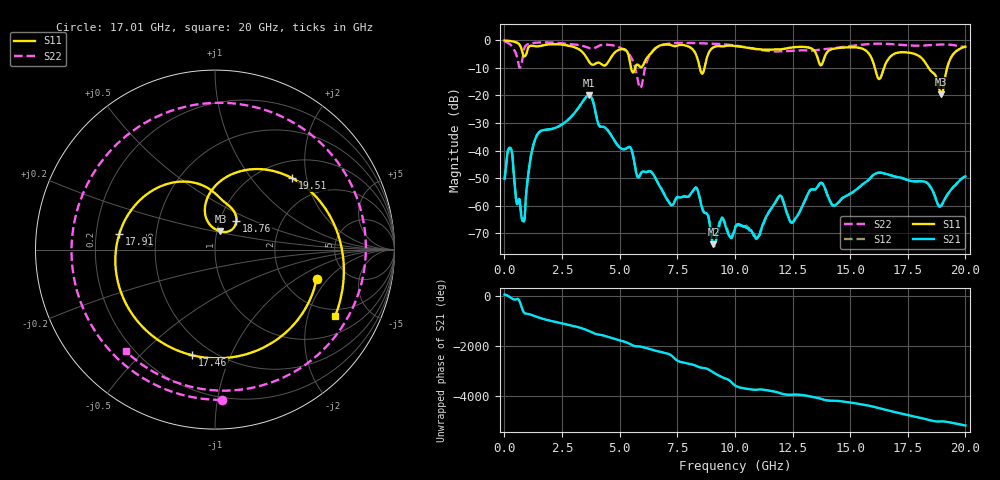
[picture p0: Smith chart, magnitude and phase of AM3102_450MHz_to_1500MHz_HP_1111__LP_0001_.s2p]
!Agilent Technologies,E8364B,MY43040894,A.07.50.67
!Agilent E8364B: A.07.50.67
!Date: Thursday, January 11, 2018 06:48:49
!Correction: S11(Full 2 Port(1,2))
!S21(Full 2 Port(1,2))
!S12(Full 2 Port(1,2))
!S22(Full 2 Port(1,2))
!S2P File: Measurements: S11, S21, S12, S22:
# Hz S  dB  R 50
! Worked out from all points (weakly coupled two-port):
!   1601 points, 10 MHz to 20 GHz, reference 50 ohm
!   highest |S21| = -19.94 dB at 3.671 GHz (marker M1); lowest = -73.9 dB at 9.068 GHz (marker M2)
!   lowest |S11| = -19.5 dB at 18.95 GHz (marker M3), VSWR 1.24, Z = 52 + j10.6 ohm
!   |S11| at or under -10 dB: 8.477 GHz to 8.683 GHz (205.6 MHz wide, 2.4 % of centre); 16.07 GHz to 16.47 GHz (396 MHz wide, 2.43 % of centre); 18.4 GHz to 19.21 GHz (809.3 MHz wide, 4.3 % of centre)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
!   |S22| runs from -17.4 to -0.4 dB; largest |S21 - S12| = 0.0017
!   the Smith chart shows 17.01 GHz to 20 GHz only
!   S11 on the Smith chart (normalised r, x): 17.01 GHz: 3.02, -1.53; 17.46 GHz: 0.39, -0.73; 17.91 GHz: 0.30, +0.07; 18.76 GHz: 1.20, +0.40; 19.51 GHz: 1.36, +1.65; 20 GHz: 1.68, -3.01
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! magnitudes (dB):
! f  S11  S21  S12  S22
! 10 MHz  -0.1  -50.3  -50.2  -0.4
! 259.9 MHz  -0.3  -39.1  -39.0  -1.5
! 809.6 MHz  -5.3  -65.5  -64.8  -5.6
! 1.409 GHz  -2.2  -34.5  -34.5  -0.9
! 3.346 GHz  -4.0  -22.9  -22.9  -1.9
! 3.671 GHz  -7.7  -19.9  -19.9  -2.8
! 5.22 GHz  -3.3  -39.5  -39.5  -3.6
! 5.895 GHz  -9.7  -48.7  -48.7  -17.4
! 6.682 GHz  -2.2  -52.1  -51.9  -2.2
! 8.331 GHz  -5.5  -53.5  -53.5  -1.0
! 9.068 GHz  -2.6  -73.9  -74.5  -1.2
! 10.01 GHz  -2.1  -68.2  -68.0  -1.9
! 12.5 GHz  -2.6  -66.1  -66.1  -3.8
! 13.34 GHz  -3.1  -54.0  -54.0  -3.8
! 16.68 GHz  -6.6  -48.7  -48.7  -1.3
! 17.01 GHz  -4.6  -49.5  -49.5  -1.5
! 17.46 GHz  -4.4  -50.6  -50.6  -1.8
! 17.91 GHz  -5.3  -51.1  -51.1  -2.0
! 18.76 GHz  -13.9  -58.5  -58.5  -1.6
! 18.95 GHz  -19.5  -60.0  -59.9  -1.5
! 19.51 GHz  -4.6  -52.9  -52.9  -1.8
! 20 GHz  -2.3  -49.4  -49.3  -2.5
